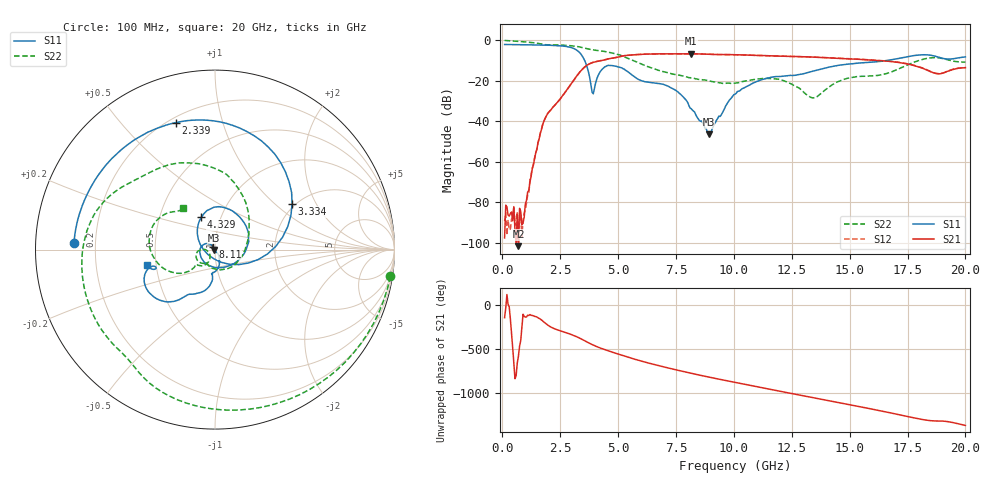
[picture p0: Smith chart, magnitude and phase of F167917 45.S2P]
!  2-Port S-parameters saved by WinCal
! VAR MeasName=S-Parameters (CALIBRATED_DATA) read from VNA (N5242A)
! VAR MeasDate=2016-11-22 9:02:01
! VAR NAME=F167917 45
! VAR FILENAME=F167917 45.S2P
! VAR DATE=2016-11-22 9:02:01
! VAR PHYS_PORTS=1,2
# Hz S DB R 50
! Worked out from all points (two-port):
!   401 points, 100 MHz to 20 GHz, reference 50 ohm
!   highest |S21| = -6.64 dB at 8.159 GHz (marker M1); lowest = -101.5 dB at 697 MHz (marker M2)
!   |S21| within 3 dB of the highest: 4.418 GHz to 15.76 GHz (11.35 GHz wide, 112 % of centre)
!   lowest |S11| = -46.3 dB at 8.906 GHz (marker M3), VSWR 1.01, Z = 49.6 - j0.258 ohm
!   |S11| at or under -10 dB: 3.557 GHz to 16.6 GHz (13.04 GHz wide, 129 % of centre)
!   |S22| runs from -28.4 to -0.1 dB; largest |S21 - S12| = 0.0048
!   S11 on the Smith chart (normalised r, x): 100 MHz: 0.12, +0.02; 2.339 GHz: 0.23, +0.71; 3.334 GHz: 1.92, +1.31; 4.329 GHz: 0.81, +0.30; 8.11 GHz: 0.97, +0.03; 20 GHz: 0.44, -0.09
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1e8  -2.09 177.3  -97.47 -147.3  -89.16 -168.6  -0.10 -8.7
6.97e8  -2.17 161.4  -101.54 135.6  -100.79 142.6  -0.53 -55.9
1.04525e9  -2.23 151.9  -78.95 -140.1  -80.20 -135.2  -0.87 -80.9
1.74175e9  -2.37 130.6  -41.70 176.9  -41.65 177.0  -2.00 -124.0
2.33875e9  -2.61 107.0  -31.14 78.6  -31.11 78.3  -2.27 -151.8
2.886e9  -3.34 74.7  -22.92 30.3  -22.92 30.2  -2.62 -178.6
3.33375e9  -6.03 30.7  -15.84 -18.9  -15.86 -18.8  -3.29 159.2
3.43325e9  -7.43 17.5  -14.57 -32.1  -14.57 -31.9  -3.54 154.5
3.93075e9  -26.37 -145.2  -10.88 -99.0  -10.84 -99.0  -4.78 135.2
4.32875e9  -14.12 112.7  -9.90 -141.1  -9.87 -141.3  -5.36 119.4
5.72175e9  -18.17 -44.6  -7.13 100.6  -7.13 100.6  -10.34 54.8
6.7665e9  -21.32 -170.7  -6.71 26.7  -6.71 26.6  -14.90 10.4
8.10975e9  -33.40 129.4  -6.66 -55.8  -6.66 -55.9  -18.44 -67.9
8.1595e9  -33.78 134.5  -6.64 -58.9  -6.65 -59.0  -18.58 -71.1
8.90575e9  -46.32 -147.5  -6.90 -101.8  -6.90 -101.9  -19.94 -106.4
1.005e10  -26.63 -62.2  -7.13 -163.4  -7.15 -163.3  -21.11 -124.7
1.179125e10  -17.92 -92.9  -7.76 106.7  -7.73 106.7  -19.04 -160.9
1.338325e10  -15.35 -95.0  -8.29 25.7  -8.24 26.0  -28.37 -154.9
1.5224e10  -11.44 -113.5  -9.28 -67.3  -9.22 -67.5  -18.10 -134.7
1.67165e10  -9.79 -123.9  -10.38 -146.3  -10.35 -146.6  -15.97 -139.3
1.8408e10  -7.25 -155.1  -15.07 125.1  -14.94 124.2  -8.80 178.6
2e10  -8.21 -167.4  -13.53 68.0  -13.46 67.3  -10.75 127.4
